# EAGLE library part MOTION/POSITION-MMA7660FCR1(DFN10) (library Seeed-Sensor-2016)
314080009
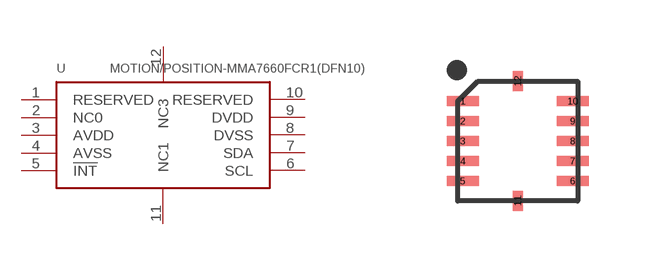
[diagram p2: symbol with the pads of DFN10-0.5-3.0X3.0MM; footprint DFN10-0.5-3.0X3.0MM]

Designator prefix U

## MOTION/POSITION-MMA7660FCR1(DFN10) (MPN: MMA7660FCR1; VALUE: MMA7660FCR1)  [DFN10-0.5-3.0X3.0MM]
1  RESERVED
2  NC0  nc
3  AVDD  pwr
4  AVSS  pwr
5  !INT
6  SCL
7  SDA
8  DVSS
9  DVDD
10  RESERVED
11  NC1  nc
12  NC3  nc

## Footprint DFN10-0.5-3.0X3.0MM (pad centres in mm)
smd 0.8 x 0.25: 1 -1.375,1; 2 -1.375,0.5; 3 -1.375,0; 4 -1.375,-0.5; 5 -1.375,-1; 6 1.375,-1; 7 1.375,-0.5; 8 1.375,0; 9 1.375,0.5; 10 1.375,1
smd 0.25 x 0.5: 11 0,-1.5; 12 0,1.5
